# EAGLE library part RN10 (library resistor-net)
RESISTOR NETWORK
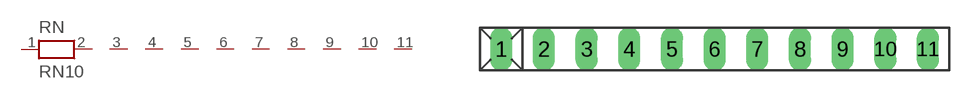
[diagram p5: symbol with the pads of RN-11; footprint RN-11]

Designator prefix RN

## RN10 (OC_FARNELL: unknown; OC_NEWARK: unknown)  [RN-11]
1  1  pas
2  2  pas
3  3  pas
4  4  pas
5  5  pas
6  6  pas
7  7  pas
8  8  pas
9  9  pas
10  10  pas
11  11  pas

## Footprint RN-11 (pad centres in mm)
RESISTOR NETWORK
drill 0.813 long: 1 -12.7,0; 2 -10.16,0; 3 -7.62,0; 4 -5.08,0; 5 -2.54,0; 6 0,0; 7 2.54,0; 8 5.08,0; 9 7.62,0; 10 10.16,0; 11 12.7,0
